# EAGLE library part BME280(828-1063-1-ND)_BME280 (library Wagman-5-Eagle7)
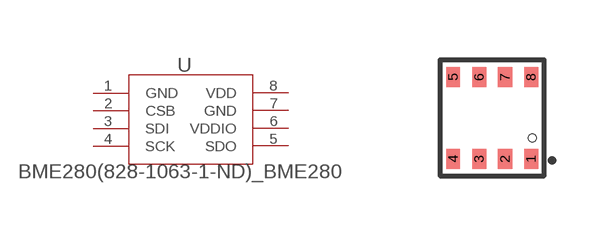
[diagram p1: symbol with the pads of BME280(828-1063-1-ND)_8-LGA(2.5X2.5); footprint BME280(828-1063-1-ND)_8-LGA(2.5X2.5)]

Designator prefix U

## BME280(828-1063-1-ND)_BME280  [BME280(828-1063-1-ND)_8-LGA(2.5X2.5)]
1  GND  pas
2  CSB  pas
3  SDI  pas
4  SCK  pas
5  SDO  pas
6  VDDIO  pas
7  GND  pas
8  VDD  pas

## Footprint BME280(828-1063-1-ND)_8-LGA(2.5X2.5) (pad centres in mm)
smd 0.35 x 0.5: 1 0.975,-1.025; 2 0.325,-1.025; 3 -0.325,-1.025; 4 -0.975,-1.025; 5 -0.975,1.025; 6 -0.325,1.025; 7 0.325,1.025; 8 0.975,1.025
